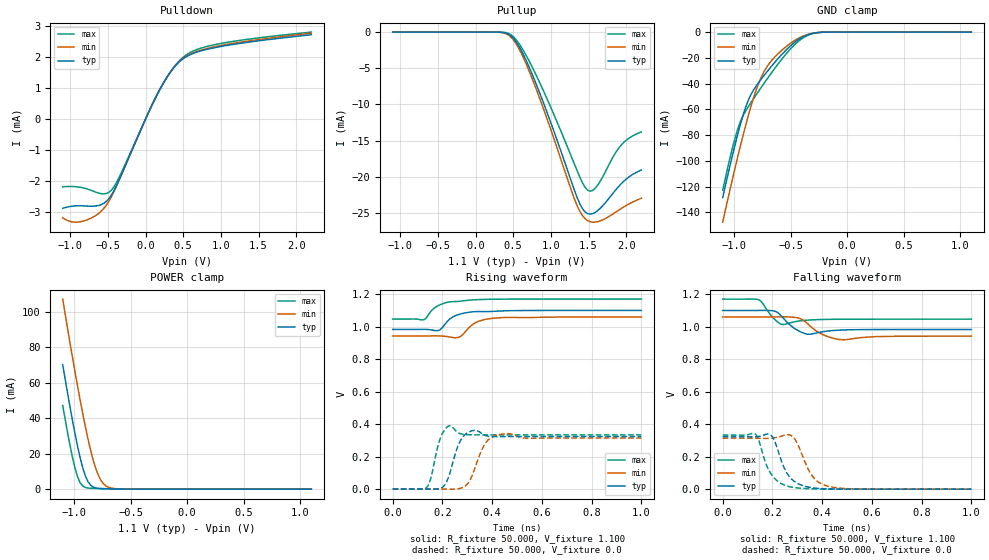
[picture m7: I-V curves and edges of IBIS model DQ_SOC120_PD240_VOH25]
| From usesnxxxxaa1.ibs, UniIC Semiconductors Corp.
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|   Model DQ_SOC120_PD240_VOH25
[Model] DQ_SOC120_PD240_VOH25
Model_type I/O
Polarity   Non-Inverting
Enable   Active-High
Vinl =  0.113V
Vinh =  0.253V
Vmeas =  0.183V
Rref =  50.000
Vref =  0.183V
C_comp   1.110pF   1.087pF   1.118pF
[Model Spec]
Vinh   0.253V   0.247V   0.265V
Vinl   0.113V   0.107V   0.125V
Vmeas   0.183V   NA   NA
Vref   0.183V   NA   NA
Rref   50.000   NA   NA
[Temperature Range]   25.000   0.125k   -40.000
[Voltage Range]   1.100V   1.060V   1.170V
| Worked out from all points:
|   slope of the pulldown table from 0 to 0.165 V, typ, clamps not added: 194 ohm
|   GND clamp passes 1 mA (typ) near -0.30 V on its own axis
|   POWER clamp passes 1 mA (typ) near -0.82 V on its own axis
|   rising waveform, R_fixture 50.000, V_fixture 1.100: 20-80 % time 63ps typ, 61.8ps min, 66.2ps max; typ from 0.983 V to 1.1 V
|   rising waveform, R_fixture 50.000, V_fixture 0.0: 20-80 % time 38.1ps typ, 47.8ps min, 29ps max; typ from 0 V to 0.323 V
|   falling waveform, R_fixture 50.000, V_fixture 1.100: 20-80 % time 44.6ps typ, 57.6ps min, 33.7ps max; typ from 1.1 V to 0.983 V
|   falling waveform, R_fixture 50.000, V_fixture 0.0: 20-80 % time 57.4ps typ, 61.3ps min, 56.5ps max; typ from 0.323 V to 0 V
[Pulldown]
|Voltage   I(typ)   I(min)   I(max)
-1.1V     -2.891mA   -3.2mA     -2.195mA
-930mV    -2.813mA   -3.341mA   -2.192mA
-760mV    -2.822mA   -3.249mA   -2.278mA
-590mV    -2.774mA   -2.987mA   -2.419mA
-454mV    -2.466mA   -2.52mA    -2.306mA
-352mV    -1.973mA   -1.987mA   -1.895mA
158mV     816.1uA    812uA      805.8uA
328mV     1.513mA    1.515mA    1.515mA
498mV     1.95mA     1.966mA    1.998mA
668mV     2.153mA    2.178mA    2.237mA
940mV     2.32mA     2.351mA    2.418mA
2.2V      2.729mA    2.779mA    2.814mA
[Pullup]
|Voltage   I(typ)   I(min)   I(max)
-1.1V     1nA        20.06nA    0A
296mV     -7.246uA   -20.98uA   -3.025uA
466mV     -481.5uA   -654.3uA   -337.8uA
568mV     -1.825mA   -2.144mA   -1.464mA
704mV     -4.678mA   -5.204mA   -3.865mA
942mV     -10.91mA   -11.79mA   -9.07mA
1.316V    -21.96mA   -23.15mA   -18.34mA
1.418V    -24.4mA    -25.34mA   -20.81mA
1.486V    -25.09mA   -26.04mA   -21.84mA
1.622V    -24.66mA   -26.19mA   -21.13mA
1.928V    -21.01mA   -24.42mA   -15.67mA
2.2V      -19.05mA   -22.95mA   -13.79mA
[GND_clamp]
|Voltage   I(typ)   I(min)   I(max)
-1.1V     -128.5mA   -147.6mA   -122.6mA
-1.008V   -93.62mA   -112mA     -87.95mA
-962mV    -77.6mA    -95.05mA   -73.96mA
-893mV    -57.36mA   -71.21mA   -60.7mA
-847mV    -48.01mA   -56.81mA   -54.36mA
-801mV    -41.47mA   -44.23mA   -48.33mA
-755mV    -36.02mA   -34.19mA   -42.41mA
-709mV    -30.9mA    -26.94mA   -36.63mA
-525mV    -12.67mA   -10.3mA    -15.49mA
-387mV    -3.615mA   -3.065mA   -4.419mA
-249mV    -281uA     -330.6uA   -301.3uA
1.1V      0A         0A         0A
[POWER_clamp]
|Voltage   I(typ)   I(min)   I(max)
-1.1V     70.27mA    107.3mA    47.25mA
-1.039V   47.68mA    83.93mA    25.86mA
-993mV    31.88mA    66.94mA    12.35mA
-970mV    24.65mA    58.72mA    7.262mA
-947mV    18.06mA    50.74mA    3.761mA
-901mV    7.73mA     35.71mA    987.1uA
-855mV    2.348mA    22.46mA    514uA
-809mV    697.3uA    11.94mA    396.5uA
-763mV    321uA      5.097mA    322.7uA
-717mV    213.8uA    1.813mA    258.1uA
-556mV    65.24uA    79.15uA    81.64uA
1.1V      0A         0A         0A
[Ramp]
| variable   typ   min   max
dV/dt_r   0.194/38.600p   0.188/48.251p   0.200/29.219p
dV/dt_f   70.211m/45.240p   70.570m/58.372p   73.998m/33.655p
R_load = 50.000
[Rising Waveform]
R_fixture= 50.000
V_fixture= 1.100
V_fixture_min= 1.060
V_fixture_max= 1.170
|time   V(typ)   V(min)   V(max)
0s        983mV      942.4mV    1.047V
122ps     983.7mV    942.5mV    1.042V
181ps     975.4mV    943.1mV    1.128V
196ps     988.3mV    942.3mV    1.138V
231ps     1.048V     936.1mV    1.153V
262ps     1.073V     932.8mV    1.156V
306ps     1.089V     993mV      1.163V
353ps     1.093V     1.037V     1.167V
443ps     1.097V     1.056V     1.169V
1ns       1.1V       1.06V      1.17V
[Rising Waveform]
R_fixture= 50.000
V_fixture= 0.0
V_fixture_min= 0.0
V_fixture_max= 0.0
|time   V(typ)   V(min)   V(max)
0s        3.571uV    28.95uV    664nV
136ps     4.93uV     79.39uV    8.309mV
152ps     -518.5uV   113.7uV    58.88mV
188ps     1.887mV    28.33uV    297.9mV
228ps     88.26mV    -963.7uV   390.2mV
264ps     271mV      1.585mV    346mV
298ps     343.7mV    26.52mV    334.8mV
366ps     334.5mV    265.3mV    333.3mV
416ps     322.2mV    330.4mV    333.3mV
1ns       323.3mV    314.2mV    333.3mV
[Falling Waveform]
R_fixture= 50.000
V_fixture= 1.100
V_fixture_min= 1.060
V_fixture_max= 1.170
|time   V(typ)   V(min)   V(max)
0s        1.1V       1.06V      1.17V
143ps     1.1V       1.06V      1.167V
206ps     1.097V     1.06V      1.05V
240ps     1.059V     1.061V     1.014V
286ps     992.5mV    1.058V     1.029V
340ps     954.5mV    1.021V     1.041V
396ps     967.5mV    956.4mV    1.045V
465ps     978.7mV    922.1mV    1.046V
612ps     982.7mV    939mV      1.047V
1ns       983mV      942.4mV    1.047V
[Falling Waveform]
R_fixture= 50.000
V_fixture= 0.0
V_fixture_min= 0.0
V_fixture_max= 0.0
|time   V(typ)   V(min)   V(max)
0s        323.3mV    314.2mV    333.3mV
133ps     322.5mV    313.6mV    337.6mV
192ps     334.9mV    313.4mV    99.58mV
210ps     291.7mV    316.6mV    64.33mV
240ps     158mV      327.8mV    30.85mV
267ps     78.97mV    334.4mV    15.77mV
292ps     43.77mV    304mV      9.105mV
357ps     9.495mV    88.03mV    2.335mV
422ps     1.925mV    18.6mV     596.9uV
1ns       8.648uV    35.81uV    3.159uV
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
